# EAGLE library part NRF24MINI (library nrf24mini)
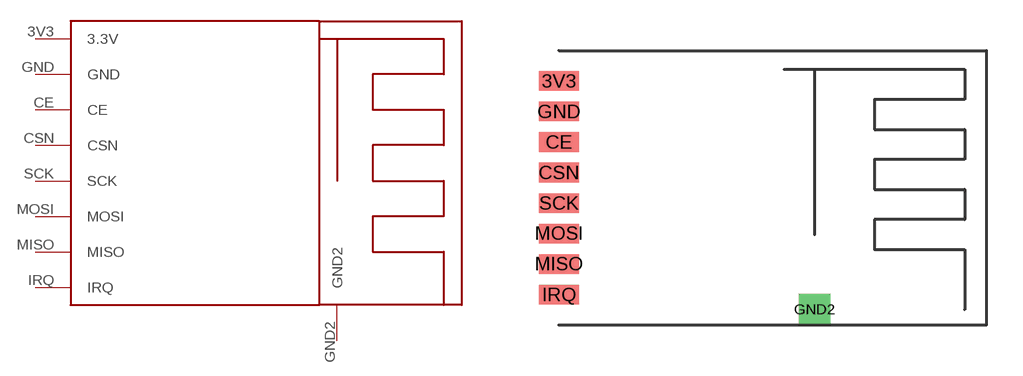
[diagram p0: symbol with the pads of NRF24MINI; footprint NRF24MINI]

Designator prefix -

## NRF24MINI  [NRF24MINI]
3V3  3.3V
CE  CE
CSN  CSN
GND  GND
GND2  GND2
IRQ  IRQ
MISO  MISO
MOSI  MOSI
SCK  SCK

## Footprint NRF24MINI (pad centres in mm)
smd 1.676 x 0.813: 3V3 0,8.89; CE 0,6.35; CSN 0,5.08; GND 0,7.62; IRQ 0,0; MISO 0,1.27; MOSI 0,2.54; SCK 0,3.81
drill 0.8 square: GND2 10.625,-0.625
